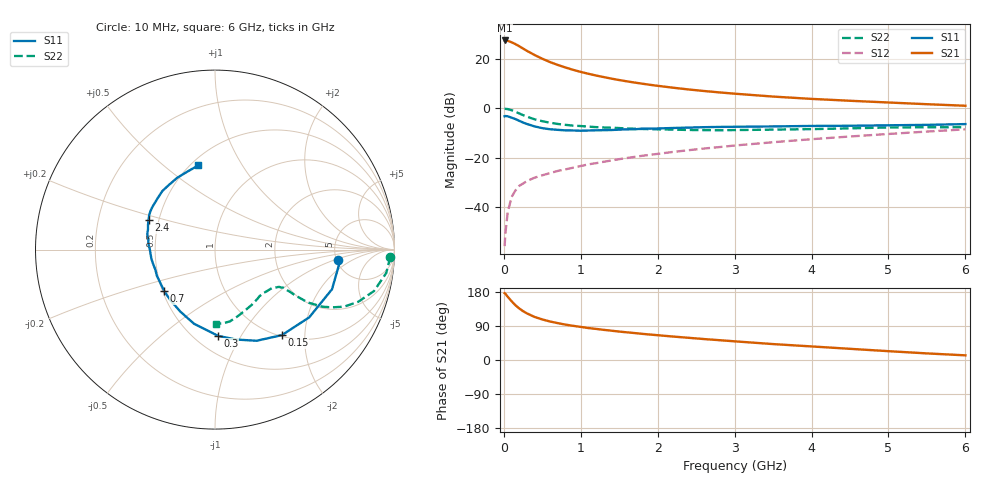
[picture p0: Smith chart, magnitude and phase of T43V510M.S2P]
! Infineon Technologies  Discrete & RF Semiconductors
! BFR182T
! Si NPN RF Bipolar Junction Transistor in SC75
! VCE = 3.5 V  IC = 10 mA
! Common Emitter S-Parameters:  October  1999
# GHz  S  MA  R  50
!  f  S11  S21  S12  S22
! GHz  MAG  ANG  MAG  ANG  MAG  ANG  MAG  ANG
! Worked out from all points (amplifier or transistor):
!   36 points, 10 MHz to 6 GHz, reference 50 ohm
!   highest |S21| = 27.5 dB at 10 MHz (marker M1)
!   |S21| within 3 dB of that: start of sweep to 234.8 MHz
!   unconditionally stable (mu >= 1): 999.4 MHz to 3.792 GHz
!   at 250 MHz: K = 0.45, MSG = 27.4 dB, |S12| = -30.5 dB
!   at 1.4 GHz: K = 1.07, MAG = 15.0 dB, |S12| = -21.2 dB
!   at 6 GHz: K = 0.84, MSG = 4.8 dB, |S12| = -8.5 dB
!   lowest NFmin = 1.50 dB at 450 MHz
!   S11 on the Smith chart (normalised r, x): 10 MHz: 5.17, -1.13; 150 MHz: 1.02, -1.53; 300 MHz: 0.64, -0.80; 700 MHz: 0.51, -0.27; 2.4 GHz: 0.44, +0.17; 6 GHz: 0.55, +0.66
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0.01  0.6888 -4.8  23.75 176.4  0.0016 74.6  0.973 -2.3
0.02  0.6976 -6.2  23.71 174.8  0.0029 96.6  0.9752 -3.1
0.05  0.6884 -18.7  23.35 166.9  0.0077 89.2  0.9629 -7.8
0.1  0.6466 -35.7  21.85 155.3  0.0158 76.6  0.9155 -14.6
0.15  0.6048 -52.0  20.06 144.6  0.0215 68.7  0.8497 -20.0
0.2  0.5582 -65.5  18.13 136.0  0.0267 66.1  0.7871 -23.8
0.25  0.5144 -76.9  16.27 128.9  0.0298 61.1  0.7267 -26.3
0.3  0.4807 -88.0  14.63 123.0  0.0335 60.1  0.6776 -28.0
0.4  0.4294 -105.8  12.04 113.6  0.0392 59.2  0.5978 -29.6
0.5  0.3958 -119.2  10.11 107.0  0.0438 58.0  0.5471 -29.7
0.6  0.3761 -131.1  8.658 101.6  0.0485 59.0  0.5097 -29.7
0.7  0.3655 -140.6  7.584 97.3  0.0536 60.0  0.4817 -29.4
0.9  0.3551 -155.8  6.028 90.2  0.0624 62.1  0.4457 -29.2
1.1  0.3542 -167.4  5.009 84.3  0.073 63.3  0.4247 -29.8
1.3  0.3601 -176.4  4.291 79.5  0.0825 64.4  0.4082 -30.7
1.6  0.3743 173.2  3.518 73.0  0.0982 65.7  0.3902 -32.7
2.2  0.3986 159.4  2.615 61.9  0.1304 66.3  0.3698 -39.0
2.4  0.406 155.8  2.412 58.6  0.1412 66.5  0.3634 -41.5
3.5  0.4286 138.4  1.729 42.0  0.2051 63.6  0.3694 -56.2
4.5  0.4425 125.4  1.421 29.5  0.2681 59.3  0.3919 -71.0
5.5  0.4615 109.2  1.211 17.4  0.3375 53.8  0.4131 -83.8
6  0.4781 101.2  1.126 12.3  0.3743 50.3  0.413 -89.0
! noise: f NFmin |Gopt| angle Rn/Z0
0.45  1.5  0.26  43  0.28
0.9  1.6  0.24  87  0.22
1.8  2.1  0.2  170  0.2
